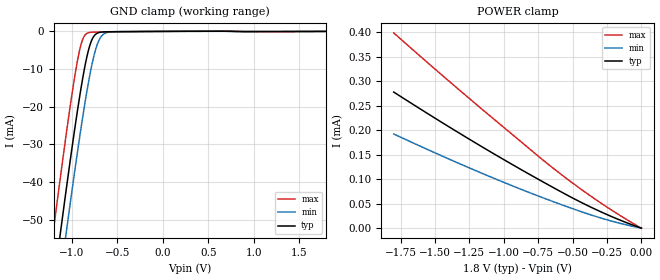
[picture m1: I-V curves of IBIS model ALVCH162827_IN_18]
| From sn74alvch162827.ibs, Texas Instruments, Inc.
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[Model]   ALVCH162827_IN_18
Model_type  Input
Vinl = 0.5775
Vinh = 1.2675
| variable   typ   min   max
C_comp   5.34pF   4.57pF   6.36pF
[Temperature Range]   40   100   -40
| Ambient temperature   25   85   -40
[Voltage range]   1.8   1.65   1.95
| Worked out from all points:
|   GND clamp passes 1 mA (typ) near -0.75 V on its own axis
[GND Clamp]
| ALVCH162827_IN_18
|   Voltage   I(typ)   I(min)   I(max)
-1.8V     -181.7mA   -192.8mA   -167.8mA
-1.205V   -67.69mA   -79.2mA    -52.93mA
-1.125V   -53mA      -64.51mA   -38.22mA
-1.06V    -41.35mA   -52.8mA    -26.68mA
-930mV    -19.52mA   -30.43mA   -6.594mA
-885mV    -12.87mA   -23.23mA   -2.305mA
-840mV    -7.196mA   -16.52mA   -586.2uA
-785mV    -2.468mA   -9.359mA   -226.7uA
-725mV    -520uA     -3.704mA   -179.8uA
-675mV    -183.7uA   -1.261mA   -163.2uA
-605mV    -102.8uA   -237.6uA   -142.7uA
1.8V      4.868pA    9.514uA    -22.72uA
[POWER Clamp]
| ALVCH162827_IN_18
|   Voltage   I(typ)   I(min)   I(max)
-1.8V     278uA      192.4uA    398.9uA
-1.2V     173.2uA    117uA      252.9uA
-645mV    83.65uA    54.61uA    123.4uA
-480mV    58.73uA    37.87uA    88.08uA
-315mV    36.04uA    22.52uA    55.28uA
-155mV    16.49uA    9.87uA     25.95uA
-16.28fV  4.868pA    8.756pA    4.988pA
